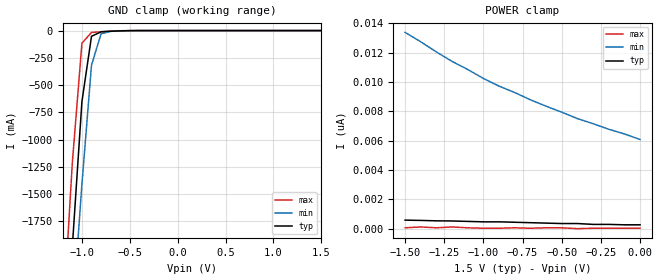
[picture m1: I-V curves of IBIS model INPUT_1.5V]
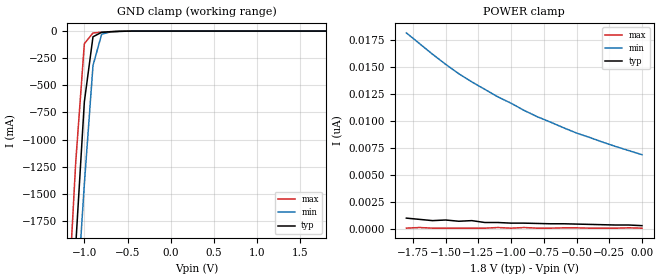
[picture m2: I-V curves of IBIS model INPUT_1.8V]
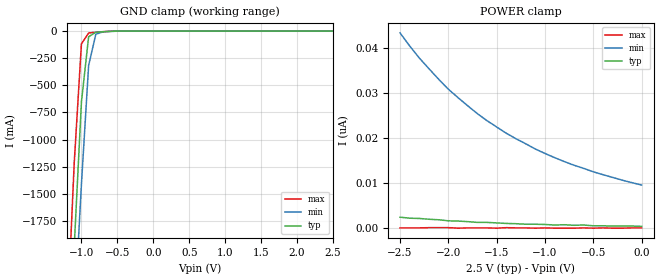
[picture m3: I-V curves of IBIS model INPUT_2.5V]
|   PERICOM SEMICONDUCTOR CORP
|   IBIS Model of PI6C10804
|   Product Family: 6C
|   SOIC 8-Pins (W) Package
[IBIS Ver] 3.2
[Comment char] |_char
[File Name] pi6c10804_w_reva.ibs
[File Rev] 1.0
[Source] File originated at Pericom Semiconductor Corp.
[Date] 06/15/16
[Disclaimer] (C) Copyright PERICOM Semiconductor Corporation
   All rights reserved
  Pericom Semiconductor Corporation hereby grants the user of
  this IBIS model a non-exclusive, nontransferable license to
  use this IBIS model under the following terms.
  This IBIS model is provided on an "AS IS" basis and Pericom
  makes absolutely no warranty with respect to the information
  contained herein. PERICOM DISCLAIMS AND CUSTOMER WAIVES ALL
  WARRANTIES, EXPRESSED OR IMPLIED, INCLUDING WARRANTIES OF
  MERCHANTABILITY OR FITNESS FOR A PARTICULAR PURPOSE. The
  entire risk as to quality and performance is with the customer.
  Accordingly, in no event shall the company be liable for any
  damages, whether in contract or tort, including any lost
  profits or other incidental, consequential, exemplary, or
  punitive damages arising out of the use or application of the
  IBIS model provided in this package. Further, Pericom reserves
  the right to make changes without notice to any product herein
  to improve reliability, function, or design. Pericom does not
  convey any license under patent rights or any other intellectual
  property rights, including those of third parties.
  The user is granted this license only to use the IBIS model
  and is not granted rights to sell, load, rent, lease or license
  the IBIS model in whole or in part, or in modified form to anyone
  other than user. User may modify the IBIS model to suit its specific
  application but rights to derivative works and such modifications
  shall belong to Pericom.
  Pericom is not obligated to provide maintenance or support
  for the licensed IBIS model.
  Contact Pericom at ATTN: APPLICATION ENGINEERING / IBIS MODELS
  1545 Barber Lane Milpitas, CA 95035 USA.
[Component] PI6C10804
[Manufacturer] Pericom Semiconductor Corp.
[Package]
| variable   typ   min   max
R_pkg   0.03093ohm   0.02906ohm   0.03279ohm
L_pkg   2.23473nH   2.04677nH   2.42269nH
C_pkg   0.22955pF   0.20548pF   0.25361pF
[Pin] signal_name   model_name   R_pin   L_pin   C_pin
1   BUF_IN   INPUT   0.03279   2.42269nH   0.25361pF
2   CLK0   OUTPUT   0.02906   2.04677nH   0.20548pF
3   CLK1   OUTPUT   0.02906   2.04677nH   0.20548pF
4   CLK2   OUTPUT   0.03279   2.26239nH   0.25361pF
5   CLK3   OUTPUT   0.03279   2.42269nH   0.25361pF
6   GND   GND   0.03279   2.42269nH   0.25361pF
7   VDD   POWER   0.02906   2.04677nH   0.20548pF
8   OE   INPUT   0.03279   2.42269nH   0.25361pF
[Model selector] INPUT
INPUT_1.5V   input pin oe/buffer_in,VDD=1,2v
INPUT_1.8V   input pin oe/buffer_in,VDD=1.8v
INPUT_2.5V   input pin oe/buffer_in,VDD=2.5v
[Model selector] OUTPUT
OUTPUT_1.5V  clock buffer output,VDD=1.5v
OUTPUT_1.8V  clock buffer output,VDD=1.8v
OUTPUT_2.5V  clock buffer output,VDD=2.5v
| Models and submodels in the file (6): INPUT_1.5V (Input), INPUT_1.8V (Input), INPUT_2.5V (Input), OUTPUT_1.5V (Output), OUTPUT_1.8V (Output), OUTPUT_2.5V (Output)
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|   Model INPUT
[Model] INPUT_1.5V
Model_type Input
Vinl = 450.00mV
Vinh = 1.0500V
| variable   typ   min   max
C_comp   1.336pF   1.335pF   1.337pF
[Voltage Range]   1.5000V   1.4250V   1.5750V
[POWER Clamp Reference]   1.5000V   1.4250V   1.5750V
[GND Clamp Reference]   0.0000V   0.0000V   0.0000V
[Temperature Range]   25   85   -40
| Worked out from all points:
|   GND clamp passes 1 mA (typ) near -0.52 V on its own axis
[GND Clamp]
| Voltage   I(typ)   I(min)   I(max)
-1.5V     -7.334A    -7.558A    -7.131A
-1.2V     -3.319A    -3.87A     -2.691A
-1.1V     -1.981A    -2.64A     -1.211A
-1V       -652mA     -1.411A    -116.3mA
-900mV    -52.46mA   -317.7mA   -17.38mA
-800mV    -11.35mA   -29.34mA   -10.41mA
-700mV    -6.003mA   -7.254mA   -5.343mA
-400mV    -60.15uA   -166.3uA   -10.59uA
1.5V      261.9pA    6.374nA    29.1pA
[POWER Clamp]
| Voltage   I(typ)   I(min)   I(max)
-1.5V     582.1pA    13.39nA    58.21pA
-1.4V     562.1pA    12.75nA    116.4pA
-1.3V     533.9pA    12.05nA    58.21pA
-1.2V     523.9pA    11.41nA    116.4pA
-1V       465.7pA    10.24nA    29.1pA
-900mV    465.7pA    9.721nA    29.1pA
-800mV    436.6pA    9.284nA    58.21pA
-700mV    407.5pA    8.789nA    29.1pA
-500mV    349.2pA    7.945nA    58.21pA
-400mV    349.2pA    7.509nA    0A
-300mV    291pA      7.16nA     29.1pA
0V        261.9pA    6.083nA    29.1pA
[Model] INPUT_1.8V
Model_type Input
Vinl = 540.00mV
Vinh = 1.2600V
| variable   typ   min   max
C_comp   1.336pF   1.335pF   1.337pF
[Voltage Range]   1.8000V   1.6500V   1.9500V
[POWER Clamp Reference]   1.8000V   1.6500V   1.9500V
[GND Clamp Reference]   0.0000V   0.0000V   0.0000V
[Temperature Range]   25   85   -40
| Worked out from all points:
|   GND clamp passes 1 mA (typ) near -0.52 V on its own axis
[GND Clamp]
| Voltage   I(typ)   I(min)   I(max)
-1.8V     -11.35A    -11.25A    -11.57A
-1.2V     -3.319A    -3.87A     -2.691A
-1.1V     -1.981A    -2.64A     -1.211A
-1V       -652mA     -1.411A    -116.3mA
-900mV    -52.46mA   -317.7mA   -17.38mA
-800mV    -11.35mA   -29.34mA   -10.41mA
-700mV    -6.003mA   -7.254mA   -5.343mA
-400mV    -60.15uA   -166.3uA   -10.59uA
1.8V      291pA      7.421nA    29.1pA
[POWER Clamp]
| Voltage   I(typ)   I(min)   I(max)
-1.8V     989.5pA    18.16nA    58.21pA
-1.7V     873.1pA    17.17nA    116.4pA
-1.6V     756.7pA    16.18nA    58.21pA
-1.5V     814.9pA    15.25nA    58.21pA
-1.4V     698.5pA    14.38nA    58.21pA
-1.3V     756.7pA    13.62nA    58.21pA
-1.2V     582.1pA    12.92nA    58.21pA
-1.1V     582.1pA    12.22nA    116.4pA
-800mV    494.8pA    10.39nA    58.21pA
-500mV    436.6pA    8.877nA    87.31pA
-200mV    349.2pA    7.625nA    58.21pA
0V        291pA      6.868nA    58.21pA
[Model] INPUT_2.5V
Model_type Input
Vinl = 750.000mV
Vinh = 1.7500V
| variable   typ   min   max
C_comp   1.336pF   1.335pF   1.337pF
[Voltage Range]   2.5000V   2.3000V   2.7000V
[POWER Clamp Reference]   2.5000V   2.3000V   2.7000V
[GND Clamp Reference]   0.0000V   0.0000V   0.0000V
[Temperature Range]   25   85   -40
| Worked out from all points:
|   GND clamp passes 1 mA (typ) near -0.52 V on its own axis
[GND Clamp]
| Voltage   I(typ)   I(min)   I(max)
-2.5V     -20.72A    -19.85A    -21.93A
-1.2V     -3.319A    -3.87A     -2.691A
-1.1V     -1.981A    -2.64A     -1.211A
-1V       -652mA     -1.411A    -116.3mA
-900mV    -52.46mA   -317.7mA   -17.38mA
-800mV    -11.35mA   -29.34mA   -10.41mA
-700mV    -6.003mA   -7.254mA   -5.343mA
-400mV    -60.15uA   -166.3uA   -10.59uA
2.5V      465.7pA    10.71nA    58.21pA
[POWER Clamp]
| Voltage   I(typ)   I(min)   I(max)
-2.5V     2.503nA    43.42nA    116.4pA
-2.4V     2.27nA     40.51nA    116.4pA
-2.3V     2.212nA    37.84nA    116.4pA
-2V       1.688nA    30.91nA    174.6pA
-1.7V     1.339nA    25.5nA     116.4pA
-1.6V     1.339nA    23.92nA    116.4pA
-1.4V     1.106nA    21.13nA    174.6pA
-1.1V     931.3pA    17.64nA    58.21pA
-800mV    814.9pA    14.84nA    58.21pA
-500mV    582.1pA    12.57nA    58.21pA
0V        465.7pA    9.633nA    116.4pA
